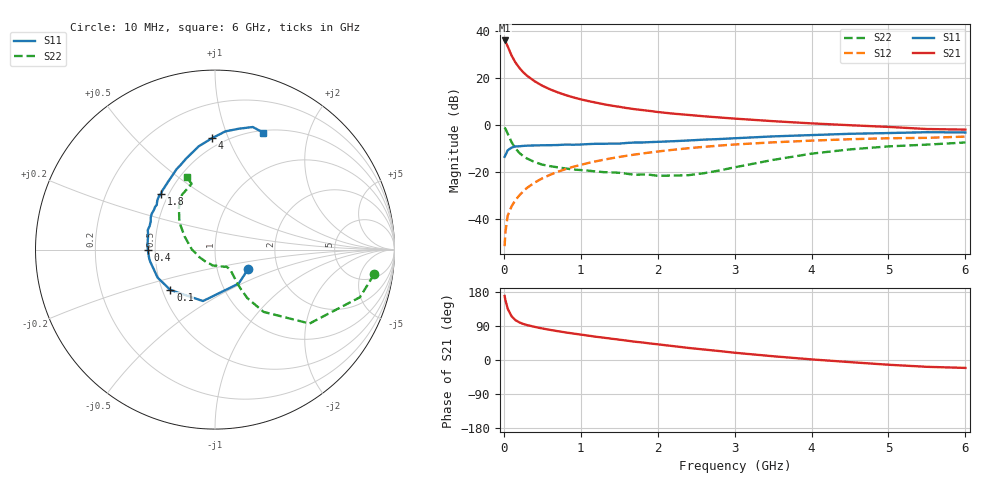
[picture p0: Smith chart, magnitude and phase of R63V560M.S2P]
! SIEMENS Small Signal Semiconductors
! BFR193
! Si NPN RF Bipolar Junction Transistor in SOT23
! VCE = 3.5 V  IC = 60 mA
! Common Emitter S-Parameters:  May  1996
# GHz  S  MA  R  50
!  f  S11  S21  S12  S22
! GHz  MAG  ANG  MAG  ANG  MAG  ANG  MAG  ANG
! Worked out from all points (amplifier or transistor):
!   36 points, 10 MHz to 6 GHz, reference 50 ohm
!   highest |S21| = 36.1 dB at 10 MHz (marker M1)
!   |S21| within 3 dB of that: start of sweep to 56.24 MHz
!   unconditionally stable (mu >= 1): 363.5 MHz to 2.029 GHz
!   at 250 MHz: K = 0.97, MSG = 25.4 dB, |S12| = -28.1 dB
!   at 1.4 GHz: K = 1.02, MAG = 10.3 dB, |S12| = -14.0 dB
!   at 6 GHz: K = 0.95, MSG = 1.5 dB, |S12| = -4.8 dB
!   S11 on the Smith chart (normalised r, x): 10 MHz: 1.42, -0.32; 100 MHz: 0.55, -0.28; 400 MHz: 0.46, -0.00; 1.8 GHz: 0.45, +0.35; 4 GHz: 0.43, +0.87; 6 GHz: 0.52, +1.36
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0.01  0.2143 -29.8  63.77 168.9  0.0027 81.2  0.8975 -8.8
0.02  0.2307 -55.2  60.88 158.5  0.0053 78.6  0.8499 -18.2
0.05  0.2944 -103.2  47.7 135.4  0.012 70.1  0.6689 -38.0
0.1  0.3355 -137.9  30.66 115.5  0.0189 70.6  0.4407 -52.0
0.15  0.3557 -154.0  21.82 105.3  0.0257 71.7  0.3249 -56.3
0.2  0.3586 -162.4  16.81 99.4  0.0322 73.1  0.2619 -56.8
0.25  0.3655 -168.4  13.57 95.3  0.0392 74.0  0.2218 -56.5
0.3  0.3699 -171.7  11.4 92.2  0.0467 74.8  0.1978 -55.6
0.4  0.374 -179.4  8.663 87.5  0.0607 75.2  0.1658 -54.2
0.5  0.377 176.2  6.955 83.2  0.0747 75.0  0.1459 -53.0
0.6  0.3787 171.1  5.836 79.5  0.0887 74.3  0.1357 -53.3
0.7  0.3814 167.6  5.032 76.1  0.1029 73.3  0.1282 -54.0
0.9  0.3873 160.0  3.945 69.9  0.1313 70.8  0.1153 -56.2
1.1  0.3996 153.7  3.278 64.2  0.1587 68.1  0.1087 -62.1
1.4  0.41 144.6  2.621 56.2  0.1995 63.8  0.1002 -71.7
1.8  0.4324 134.0  2.112 46.2  0.2521 57.6  0.0901 -91.7
2.2  0.4597 124.7  1.776 36.7  0.302 51.5  0.0856 -120.3
3.5  0.5824 99.0  1.227 9.9  0.4353 30.8  0.1842 156.7
4  0.6207 91.6  1.101 1.6  0.4732 23.7  0.2501 142.5
4.5  0.6613 85.0  1.006 -5.6  0.507 16.6  0.3082 130.7
5.5  0.7146 72.9  0.835 -18.0  0.5422 2.9  0.3892 109.5
6  0.7054 67.6  0.812 -20.9  0.5762 -1.1  0.432 111.5
